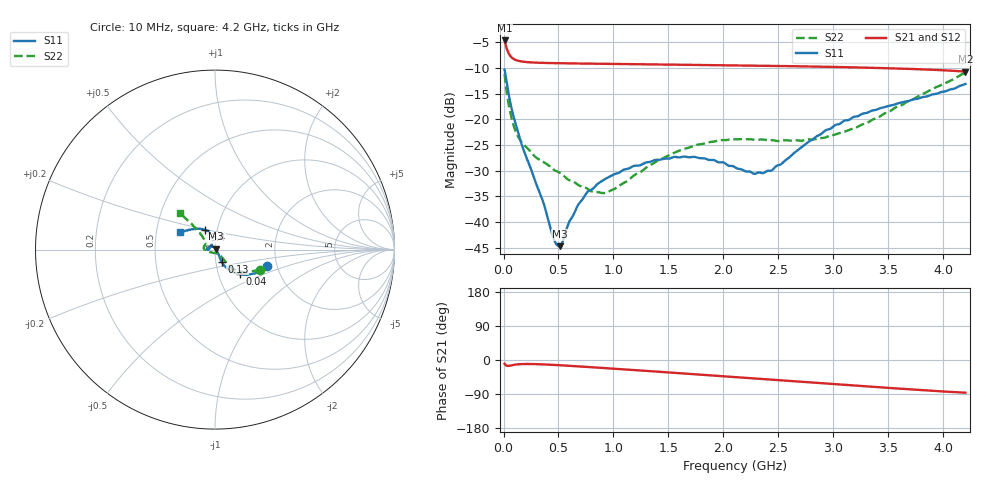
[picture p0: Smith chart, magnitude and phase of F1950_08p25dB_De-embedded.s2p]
! Integrated Device Technology
! Corporate Headquarters
! 6024 Silver Creek Valley Road
! San Jose, CA 95138  USA
! Phone:  1-408-284-8200
! Toll Free:  1-800-223-1366
! Webpage:  http://www.idt.com/
! Timing and RF Division
! 515 Groton Road, Suite 102
! Westford, MA 01886-6024
! Device:  F1950
! Description: 7-bit 0.25 dB Digital Step Attenuator
! Frequency:  150.0 -  4000.00 MHz
! Package:  4x4 mm Thin QFN Plastic Package: 24 pin
! Ports:  2 RF, 12 DC
!  Pin  1  = D0
!  Pin  2  = VDD
!  Pin  3  = Vmode
!  Pin  4  = GND
!  Pin  5  = RF1  =  Port 1
!  Pin  6  = GND
!  Pin  7  = GND
!  Pin  8  = GND
!  Pin  9  = GND
!  Pin 10  = GND
!  Pin 11  = GND
!  Pin 12  = GND
!  Pin 13  = GND
!  Pin 14  = RF2  =  Port 2
!  Pin 15  = GND
!  Pin 16  = LE
!  Pin 17  = CLK
!  Pin 18  = DATE
!  Pin 19  = D6
!  Pin 20  = D5
!  Pin 21  = D4
!  Pin 22  = D3
!  Pin 23  = D2
!  Pin 24  = D1
! State:  33
! Atten State:  8.25 dB
! Voltage:  +5.00 Volts
! Current:  Not Measured mA
! Data:  The device was measured on a the F195X evaluation board which has
!  individual transmission lines to the RF pins.  Data was collected
!  using a calibrated network analyzer.  The evaluation board was
!  de-embedded using a TRL calibration technique.
!  The reference plane is the edge of the package pin.
! Misc:  Board 2019
!  Action Tracker AT0250
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# GHz S dB R 50
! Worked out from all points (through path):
!   420 points, 10 MHz to 4.2 GHz, reference 50 ohm
!   highest |S21| = -4.68 dB at 10 MHz (marker M1); lowest = -10.7 dB at 4.2 GHz (marker M2)
!   group delay of S21, straight-line fit = 54.1 ps
!   lowest |S11| = -44.7 dB at 510 MHz (marker M3), VSWR 1.01, Z = 50.3 + j0.472 ohm
!   |S11| at or under -10 dB: start of sweep to end of sweep
!   |S22| runs from -34.4 to -10.9 dB; largest |S21 - S12| = 0.00046
!   S11 on the Smith chart (normalised r, x): 10 MHz: 1.77, -0.35; 40 MHz: 1.26, -0.36; 130 MHz: 1.07, -0.14; 3.4 GHz: 0.87, +0.20; 4.2 GHz: 0.66, +0.14
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0.01  -10.37 -17.3  -4.68 -10.0  -4.67 -10.0  -11.19 -23.7
0.04  -14.25 -44.9  -6.86 -15.6  -6.86 -15.6  -16.28 -46.4
0.08  -18.51 -57.9  -8.09 -13.6  -8.09 -13.6  -20.32 -49.8
0.13  -22.39 -61.5  -8.61 -11.5  -8.61 -11.5  -23.29 -48.1
0.28  -31.52 -51.2  -8.98 -10.8  -8.97 -10.8  -27.12 -47.8
0.36  -36.05 -37.3  -9.04 -11.6  -9.04 -11.6  -28.27 -49.4
0.45  -42.82 -1.4  -9.08 -12.8  -9.08 -12.8  -29.69 -51.2
0.51  -44.67 53.3  -9.10 -13.8  -9.10 -13.8  -30.36 -54.7
0.6  -39.82 100.7  -9.13 -15.3  -9.13 -15.3  -31.85 -60.8
0.71  -35.79 119.6  -9.16 -17.3  -9.16 -17.3  -33.07 -72.2
0.77  -34.00 125.1  -9.18 -18.5  -9.18 -18.5  -33.61 -79.9
0.94  -31.42 140.4  -9.23 -21.7  -9.22 -21.7  -34.20 -111.2
1.41  -27.87 170.0  -9.34 -30.9  -9.34 -30.9  -27.92 -164.8
1.74  -27.31 -179.1  -9.43 -37.5  -9.42 -37.6  -25.07 -178.1
2.11  -29.38 174.4  -9.53 -45.1  -9.53 -45.1  -23.91 171.4
2.28  -30.60 155.3  -9.58 -48.5  -9.57 -48.6  -23.98 166.9
2.43  -30.01 133.4  -9.62 -51.5  -9.62 -51.6  -24.05 162.6
2.81  -23.92 105.7  -9.74 -59.4  -9.74 -59.5  -23.95 148.0
3.1  -20.27 108.8  -9.86 -65.5  -9.86 -65.5  -22.44 139.7
3.4  -18.06 117.9  -10.02 -71.6  -10.01 -71.7  -19.72 134.1
3.51  -17.34 122.3  -10.08 -73.8  -10.07 -73.9  -18.50 132.9
4.2  -13.14 153.4  -10.72 -86.3  -10.72 -86.4  -10.94 134.0
